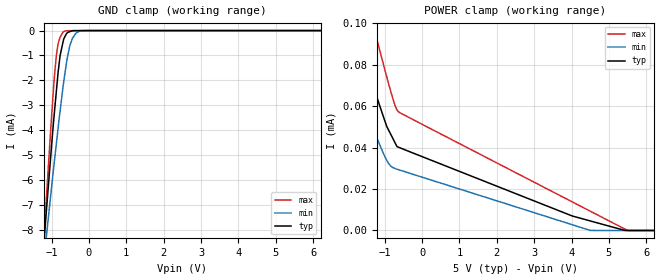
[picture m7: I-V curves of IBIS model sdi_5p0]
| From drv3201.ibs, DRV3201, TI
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|   sdi_5p0 Model
[Model]   sdi_5p0
Model_type   Input
Vinl = 1.5
Vinh = 3.5
|   typ   min   max
|   (nom PVT)   (fast PVT)   (slow PVT)
C_comp   4.496e-13   4.401e-13   4.837e-13
| Where nom  PVT is Nominal Process, 5V, 27C
|   Fast PVT is Strong Process,  5.5V, -40C
|   Slow PVT is Weak Process,   4.5V, 150C
[Voltage Range]   5   4.5   5.5
|Junction Temperature
[Temperature Range]   27   150   -40
[Power Clamp Reference]   5   4.5   5.5
[GND Clamp Reference]   0   0   0
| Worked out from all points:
|   GND clamp passes 1 mA (typ) near -0.77 V on its own axis
[GND Clamp]
|   Voltage   I(typ)   I(min)   I(max)
-5V       -87.87mA   -68.71mA   -109.8mA
-1.21V    -8.666mA   -9.333mA   -8.566mA
-1.139V   -7.275mA   -8.289mA   -6.784mA
-1.083V   -6.236mA   -7.507mA   -5.443mA
-940.5mV  -3.586mA   -5.491mA   -2.212mA
-869mV    -2.418mA   -4.533mA   -993.9uA
-770mV    -1.004mA   -3.23mA    -267.4uA
-682mV    -394.4uA   -2.153mA   -45.39uA
-513mV    -44.3uA    -626.8uA   -5.679uA
-346.5mV  -3.19uA    -105.8uA   -3.233uA
-202.5mV  -1.865uA   -6.986uA   -1.889uA
10V       0A         0A         0A
[POWER Clamp]
|   Voltage   I(typ)   I(min)   I(max)
-5V       282.9uA    230.2uA    362.8uA
-2.439V   134.6uA    103.7uA    179.4uA
-1.903V   103.7uA    77.6uA     141.3uA
-1.809V   98.4uA     73.02uA    134.6uA
-1.373V   73.62uA    52.27uA    103.8uA
-1.228V   65.62uA    45.65uA    93.82uA
-936mV    50uA       33.64uA    73.69uA
-706.5mV  41.85uA    29.83uA    59.76uA
-610.5mV  40.1uA     29.27uA    57.07uA
4.495V    4.638uA    28.64nA    9.373uA
5.5V      0A         0A         0A
10V       0A         0A         0A
